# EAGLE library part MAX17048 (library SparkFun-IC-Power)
Micropower 1-Cell Li+ ModelGauge SparkFun Products Qduino Mini (DEV-13614)
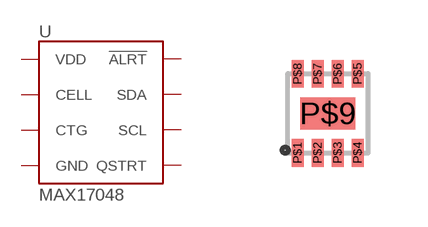
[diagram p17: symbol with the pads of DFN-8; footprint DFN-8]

Designator prefix -

## MAX17048DFN8 (PROD_ID: IC-12551; VALUE: MAX17048)  [DFN-8]
P$1  CTG  in
P$2  CELL  in
P$3  VDD
P$4  GND
P$5  !ALRT
P$6  QSTRT
P$7  SCL  out
P$8  SDA  in
P$9  GND

## Footprint DFN-8 (pad centres in mm)
Now follows http://pdfserv.maximintegrated.com/land_patterns/90-0065.PDF Pasted was reduced by 40% width on the center ground pad, and some amount on the other 8. Stop mask extends 135 µm wider than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
smd 0.3 x 0.7: P$1 -0.75,-0.99; P$2 -0.25,-0.99; P$3 0.25,-0.99; P$4 0.75,-0.99; P$5 0.75,0.99; P$6 0.25,0.99; P$7 -0.25,0.99; P$8 -0.75,0.99
smd 1.38 x 0.8: P$9 0,0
